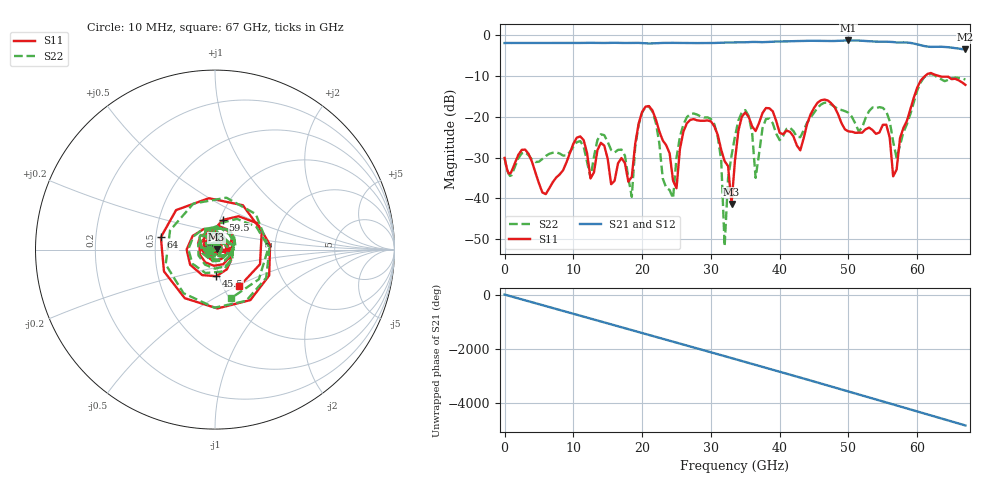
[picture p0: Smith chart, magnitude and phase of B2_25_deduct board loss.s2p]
!Keysight Technologies,N5247B,MY61255065,A.16.20.04
!Date: Sunday, September 03, 2023 21:52:06
!Correction: S11(C  2-Port  )
!S21(C  2-Port  )
!S12(C  2-Port  )
!S22(C  2-Port  )
!S2P File: Measurements: S11, S21, S12, S22:
!Deduct Board Loss
# Hz S  dB  R 50
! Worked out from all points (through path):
!   142 points, 10 MHz to 67 GHz, reference 50 ohm
!   highest |S21| = -1.32 dB at 50 GHz (marker M1); lowest = -3.5 dB at 67 GHz (marker M2)
!   lowest |S11| = -41.4 dB at 33 GHz (marker M3), VSWR 1.02, Z = 50.9 + j0.116 ohm
!   |S11| at or under -10 dB: start of sweep to 61.16 GHz; 63.13 GHz to end of sweep
!   |S22| runs from -51.7 to -9.5 dB; largest |S21 - S12| = 0.0035
!   S11 on the Smith chart (normalised r, x): 10 MHz: 0.94, -0.01; 45.5 GHz: 0.97, -0.29; 59.5 GHz: 1.03, +0.35; 64 GHz: 0.53, +0.08; 67 GHz: 1.19, -0.52
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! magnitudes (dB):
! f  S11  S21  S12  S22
! 10 MHz  -30.1  -1.9  -1.9  -30.1
! 6 GHz  -39.0  -1.9  -1.9  -29.6
! 11.5 GHz  -25.7  -1.9  -1.9  -27.3
! 18.5 GHz  -34.7  -1.9  -1.9  -39.7
! 20 GHz  -18.8  -2.0  -2.0  -19.0
! 22.5 GHz  -23.6  -2.0  -2.0  -26.5
! 24.5 GHz  -35.7  -1.9  -1.9  -40.0
! 26.5 GHz  -21.6  -2.0  -2.0  -20.1
! 30.5 GHz  -22.4  -1.9  -1.9  -21.9
! 31.5 GHz  -28.1  -1.9  -1.9  -30.7
! 32 GHz  -30.9  -1.8  -1.8  -51.7
! 33 GHz  -41.4  -1.8  -1.8  -29.6
! 34 GHz  -23.4  -1.8  -1.8  -20.9
! 36.5 GHz  -23.5  -1.7  -1.7  -35.0
! 38 GHz  -17.9  -1.7  -1.7  -20.6
! 45 GHz  -17.8  -1.4  -1.4  -19.0
! 45.5 GHz  -16.6  -1.4  -1.4  -17.8
! 50 GHz  -23.6  -1.3  -1.3  -19.0
! 56 GHz  -25.1  -1.7  -1.7  -21.1
! 59.5 GHz  -15.3  -2.1  -2.1  -16.4
! 64 GHz  -10.2  -2.9  -2.9  -11.3
! 67 GHz  -12.2  -3.5  -3.5  -10.9
